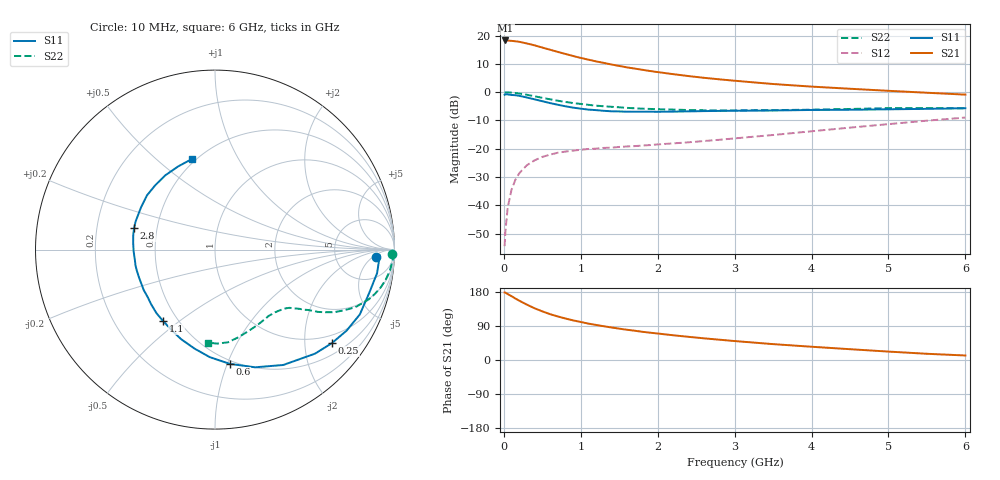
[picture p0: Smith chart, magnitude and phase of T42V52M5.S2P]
! Infineon Technologies  Discrete & RF Semiconductors
! BFR182T
! Si NPN RF Bipolar Junction Transistor in SC75
! VCE = 2.5 V  IC = 2.5 mA
! Common Emitter S-Parameters:  October  1999
# GHz  S  MA  R  50
!  f  S11  S21  S12  S22
! GHz  MAG  ANG  MAG  ANG  MAG  ANG  MAG  ANG
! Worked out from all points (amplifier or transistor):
!   36 points, 10 MHz to 6 GHz, reference 50 ohm
!   highest |S21| = 18.3 dB at 20 MHz (marker M1)
!   |S21| within 3 dB of that: start of sweep to 564.8 MHz
!   unconditionally stable (mu >= 1): 1.828 GHz to 4.262 GHz
!   at 250 MHz: K = 0.16, MSG = 22.4 dB, |S12| = -27.2 dB
!   at 1.4 GHz: K = 0.85, MSG = 14.7 dB, |S12| = -19.6 dB
!   at 6 GHz: K = 0.83, MSG = 4.1 dB, |S12| = -9.0 dB
!   lowest NFmin = 1.10 dB at 450 MHz
!   S11 on the Smith chart (normalised r, x): 10 MHz: 16, -7; 250 MHz: 0.78, -2.66; 600 MHz: 0.47, -1.02; 1.1 GHz: 0.42, -0.44; 2.8 GHz: 0.37, +0.11; 6 GHz: 0.48, +0.66
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0.01  0.9001 -2.7  8.134 178.2  0.0019 75.1  0.9879 -1.4
0.02  0.919 -2.0  8.2 177.8  0.0034 97.8  0.991 -1.4
0.05  0.9124 -8.3  8.17 174.0  0.0091 89.3  0.9915 -3.4
0.1  0.8925 -15.7  8.064 168.4  0.0189 82.6  0.9818 -6.7
0.15  0.8841 -24.1  7.936 162.2  0.0283 77.1  0.9665 -9.9
0.25  0.8343 -38.6  7.516 151.2  0.0437 69.7  0.9236 -15.6
0.3  0.8043 -46.1  7.249 146.0  0.0512 66.3  0.8995 -18.0
0.4  0.7469 -59.4  6.72 136.4  0.0625 59.8  0.8457 -22.3
0.5  0.6928 -71.2  6.146 128.4  0.0718 55.7  0.7944 -25.2
0.6  0.6416 -82.7  5.628 121.0  0.0787 52.0  0.7484 -27.8
0.7  0.5998 -92.8  5.156 115.0  0.085 49.3  0.7064 -29.6
0.8  0.5632 -101.7  4.739 109.5  0.0892 46.9  0.6724 -31.1
0.9  0.5333 -110.8  4.357 104.6  0.0926 45.6  0.642 -32.1
1.1  0.4919 -126.0  3.752 96.0  0.0992 43.8  0.5969 -34.1
1.3  0.4685 -139.3  3.291 89.0  0.1036 43.4  0.5631 -35.7
1.6  0.4519 -156.0  2.745 79.8  0.1098 44.1  0.5281 -37.9
2.2  0.4535 -178.9  2.083 65.3  0.1245 48.6  0.4919 -43.9
2.8  0.4663 165.1  1.687 53.6  0.1441 53.2  0.4751 -51.3
3.5  0.4745 150.4  1.394 41.9  0.1751 57.3  0.482 -60.4
4.5  0.4892 133.0  1.149 28.5  0.2364 58.7  0.5048 -74.7
5.5  0.507 113.8  0.977 16.4  0.3136 55.8  0.524 -88.5
6  0.5204 104.5  0.905 11.9  0.3558 52.7  0.5198 -94.6
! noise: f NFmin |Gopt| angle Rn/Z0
0.45  1.1  0.39  29  0.35
0.9  1.2  0.37  59  0.28
1.8  1.8  0.28  128  0.2
